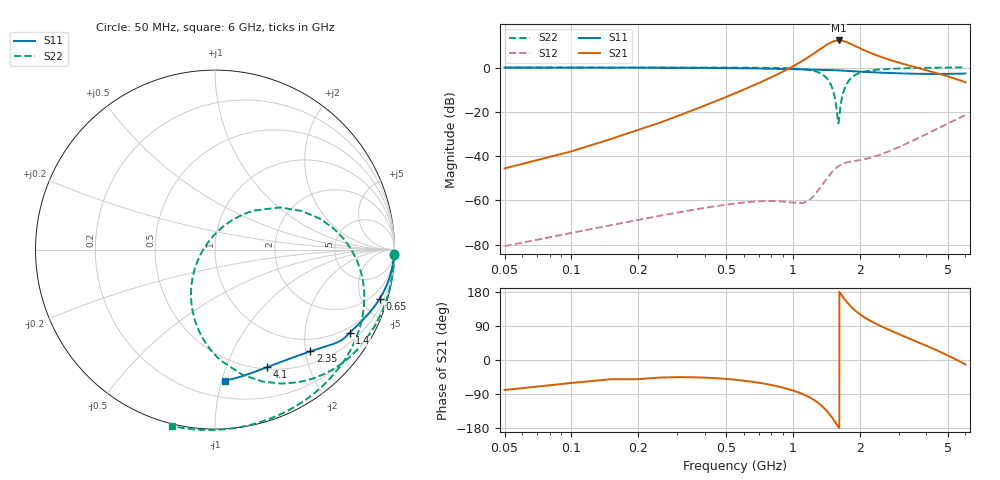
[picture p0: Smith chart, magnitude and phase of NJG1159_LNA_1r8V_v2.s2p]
! Created Mon Mar 05 15:35:43 2018
# hz S ma R 50
! 2 Port Network Data from SP6.SP block
! freq  magS11  angS11  magS21  angS21  magS12  angS12  magS22  angS22
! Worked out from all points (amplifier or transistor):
!   414 points, 50 MHz to 6 GHz, reference 50 ohm
!   highest |S21| = 12.2 dB at 1.611 GHz (marker M1)
!   |S21| within 3 dB of that: 1.37 GHz to 1.955 GHz (585.7 MHz wide, 35.2 % of centre)
!   unconditionally stable (mu >= 1): 476.8 MHz to 2.589 GHz
!   at 1.442 GHz: K = 7.11, MAG = 18.5 dB, |S12| = -49.3 dB
!   at 1.58 GHz: K = 5.46, MAG = 18.3 dB, |S12| = -45.0 dB
!   at 6 GHz: K = -0.79, MSG = 7.4 dB, |S12| = -21.4 dB
!   lowest NFmin = 0.12 dB at 100 MHz
!   S11 on the Smith chart (normalised r, x): 50 MHz: 11, -83; 650 MHz: 1.01, -6.67; 1.4 GHz: 0.79, -3.33; 2.35 GHz: 0.73, -2.10; 4.1 GHz: 0.52, -1.41; 6 GHz: 0.33, -1.03
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5e7  0.9968 -1.4  0.005279 -79.1  9.274e-05 87.9  1 -1.7
1.5e8  0.9946 -4.1  0.02414 -50.9  0.0002752 85.1  0.9997 -5.0
2.5e8  0.9903 -6.7  0.05656 -46.4  0.0004489 82.4  0.9989 -8.4
5.5e8  0.9673 -14.3  0.2644 -52.1  0.0008529 72.8  0.9934 -19.3
6.5e8  0.9573 -16.7  0.3775 -57.2  0.0009294 68.6  0.9897 -23.3
1e9  0.9186 -24.2  1.063 -80.5  0.0008994 34.9  0.9522 -41.3
1.15e9  0.9029 -27.1  1.608 -94.4  0.0009283 -8.4  0.9017 -52.9
1.25e9  0.8938 -29.0  2.115 -106.2  0.001315 -43.8  0.8348 -63.4
1.4e9  0.8827 -31.8  3.115 -130.2  0.002821 -84.1  0.6214 -86.7
1.402e9  0.8826 -31.9  3.129 -130.6  0.002849 -84.5  0.6171 -87.1
1.496e9  0.8755 -33.8  3.753 -150.7  0.004304 -106.1  0.3693 -109.6
1.557e9  0.8692 -35.2  4.011 -165.2  0.005274 -119.8  0.1694 -133.7
1.611e9  0.862 -36.3  4.086 -178.0  0.006018 -131.2  0.06195 115.3
1.687e9  0.8502 -37.8  3.962 165.2  0.00678 -145.0  0.2751 48.4
1.698e9  0.8485 -38.0  3.928 163.0  0.006864 -146.8  0.3051 45.2
1.7e9  0.8481 -38.0  3.921 162.6  0.006878 -147.1  0.3105 44.6
1.85e9  0.8257 -40.4  3.304 137.9  0.0076 -164.5  0.6073 16.6
2.05e9  0.8025 -43.1  2.587 116.7  0.008304 -174.9  0.7856 -3.3
2.35e9  0.7768 -46.8  1.94 96.7  0.00991 -179.6  0.8861 -20.5
2.75e9  0.7522 -51.5  1.478 78.1  0.01324 178.9  0.936 -35.1
4.1e9  0.7172 -66.0  0.8382 35.0  0.03329 172.9  0.9869 -68.0
6e9  0.7326 -85.6  0.4647 -11.8  0.08502 157.7  1.012 -103.8
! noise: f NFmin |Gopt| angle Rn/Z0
5e+07  0.5974  0.965  2.326  3.902
1.418e+09  0.5459  0.8235  33.68  0.5654
1.464e+09  0.5583  0.8191  34.71  0.56
1.51e+09  0.5709  0.8146  35.75  0.5546
1.556e+09  0.5838  0.8101  36.78  0.5492
1.602e+09  0.597  0.8055  37.81  0.5438
1.648e+09  0.6104  0.8009  38.84  0.5385
1.694e+09  0.624  0.7961  39.86  0.5333
3.7e+09  1.478  0.5521  77.97  0.36
6e+09  3.541  0.4353  84.89  0.6889
